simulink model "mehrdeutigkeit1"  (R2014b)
settings: Solver=ode45  StartTime=0.0  StopTime=0.01  MaxStep=1e-5  RelTol=1e-3
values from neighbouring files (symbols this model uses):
  f1 = 10    [DA_wandler_spektr_1.m]    (also in DA_wandler_spektr_2.m; fourier_reihe1.m = 100; fourier_reihe2.m = 100; mehrdeutigkeit_1.m = -200)
  f2 = 40    [DA_wandler_spektr_1.m]    (also in DA_wandler_spektr_2.m; fourier_reihe1.m = ',num2str(f2),     ' Hz; fourier_reihe2.m = 200; mehrdeutigkeit_1.m = 1800)
  fs = 4000    [abtast_rate_1.m]    (also in ad_test_12.m = ',     num2str(fs),'; ad_test_2.m = ',     num2str(fs),'; ad_test_3.m = ',     num2str(fs),'; DA_wandler_spektr_1.m = 100)
  N = 4*1024    (= 4096)    [ad_test_12.m]    (also in ad_test_2.m; ad_test_3.m; DA_wandler_spektr_1.m = 1000; DA_wandler_spektr_2.m = 1024)
  phi1 = pi/3    (= 1.0471975512)    [fourier_reihe1.m]    (also in fourier_reihe2.m; leakage_3.m; leakage_4.m; mehrdeutigkeit_1.m = 3.14159265359)
  phi2 = pi/4    (= 0.785398163397)    [fourier_reihe1.m]    (also in fourier_reihe2.m; leakage_3.m = 0.628318530718; leakage_4.m = 0.628318530718; mehrdeutigkeit_1.m = 3.14159265359)
  wp = sum(hanning(N).^2)    [mehrdeutigkeit_1.m]    (also in spektr_pulse_1.m)
undefined symbols (not defined in the file or in its folder): get
libraries: dspspect3 x1, dspsnks4 x1, dspsigops x1

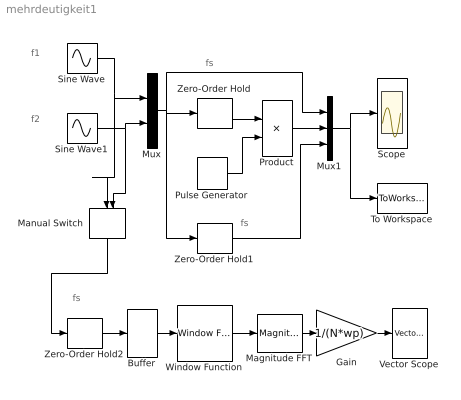
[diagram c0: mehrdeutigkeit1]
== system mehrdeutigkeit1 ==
  note: fs
  note: fs
  note: fs
  note: f2
  note: f1
  Buffer : Buffer  N=N  TreatMby1Signals=One channel
  Gain : Gain  Gain=1/(N*wp)
  Magnitude FFT : dspspect3/Magnitude FFT  mag_or_magsq=Magnitude squared  FFTImplementation=Auto  fftLenInherit=off  fftsize=256  WrapInput=on
  Manual Switch : ManualSwitch
  Mux : Mux  Inputs=2
  Mux1 : Mux  Inputs=3
  Product : Product
  Pulse Generator : DiscretePulseGenerator  PulseType=Time based  Period=1/fs  PulseWidth=15
  Scope : Scope
  Sine Wave : Sin  Frequency=2*pi*f1  Phase=phi1  SampleTime=0
  Sine Wave1 : Sin  Frequency=2*pi*f2  Phase=phi2  SampleTime=0
  To Workspace : ToWorkspace  VariableName=y  SaveFormat=Timeseries  SampleTime=-1
  Vector Scope : dspsnks4/Vector Scope  ScopeProperties=on  Domain=Frequency  HorizSpan=1  DisplayProperties=off  AxisGrid=on  Memory=off  FrameNumber=on  AxisLegend=off  AxisZoom=off  OpenScopeAtSimStart=on  OpenScopeImmediately=off  FigPos=get(0,'defaultfigureposition')  AxisProperties=off  XUnits=Hertz  XRange=[0...Fs]  InheritXIncr=off  XIncr=1/fs  XLabel=Time  XLimit=User-defined  XMin=0  XMax=1000  XStart=0  YUnits=dB  YLabel=Leistung in dB  LineProperties=off  XAxisParamsVer=6.9
  Window Function : dspsigops/Window Function  winmode=Apply window to input  wintype=Hanning  sampmode=Continuous  samptime=1  N=64  Rs=50  beta=10  winsamp=Symmetric  UserWindow=hamming  OptParams=off  UserParams={'symmetric'}  RowConvenienceOn=on  dataType=double  isSigned=on  wordLen=16  udDataType=sfix(16)  fracBitsMode=Best precision  numFracBits=15  roundingMode=Floor  overflowMode=off  numSidelobes=4  sidelobeLevel=-30
  Zero-Order Hold : ZeroOrderHold  SampleTime=1/fs
  Zero-Order Hold1 : ZeroOrderHold  SampleTime=1/fs
  Zero-Order Hold2 : ZeroOrderHold  SampleTime=1/fs
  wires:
  Zero-Order Hold/1 -> Product/1
  Mux/1 -> Zero-Order Hold1/1, Mux1/1, Zero-Order Hold/1
  Sine Wave1/1 -> Manual Switch/2, Mux/2
  Sine Wave/1 -> Manual Switch/1, Mux/1
  Product/1 -> Mux1/2
  Mux1/1 -> Scope/1, To Workspace/1
  Pulse Generator/1 -> Product/2
  Zero-Order Hold1/1 -> Mux1/3
  Buffer/1 -> Window Function/1
  Window Function/1 -> Magnitude FFT/1
  Magnitude FFT/1 -> Gain/1
  Gain/1 -> Vector Scope/1
  Zero-Order Hold2/1 -> Buffer/1
  Manual Switch/1 -> Zero-Order Hold2/1
